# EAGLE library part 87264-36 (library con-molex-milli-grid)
RECEPTACAL
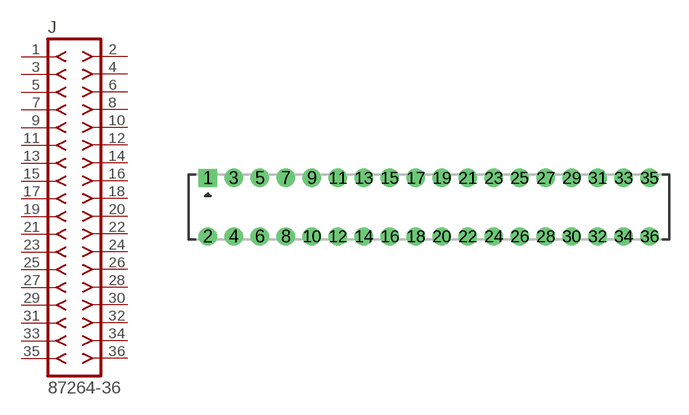
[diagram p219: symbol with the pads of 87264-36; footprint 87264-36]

Designator prefix J

## 87264-36  [87264-36]
1  1  pas
2  2  pas
3  3  pas
4  4  pas
5  5  pas
6  6  pas
7  7  pas
8  8  pas
9  9  pas
10  10  pas
11  11  pas
12  12  pas
13  13  pas
14  14  pas
15  15  pas
16  16  pas
17  17  pas
18  18  pas
19  19  pas
20  20  pas
21  21  pas
22  22  pas
23  23  pas
24  24  pas
25  25  pas
26  26  pas
27  27  pas
28  28  pas
29  29  pas
30  30  pas
31  31  pas
32  32  pas
33  33  pas
34  34  pas
35  35  pas
36  36  pas

## Footprint 87264-36 (pad centres in mm)
RECEPTACAL Dual Row, Side Entry
drill 0.914 square: 1 -17,2.25
drill 0.914: 2 -17,-2.25; 3 -15,2.25; 4 -15,-2.25; 5 -13,2.25; 6 -13,-2.25; 7 -11,2.25; 8 -11,-2.25; 9 -9,2.25; 10 -9,-2.25; 11 -7,2.25; 12 -7,-2.25; 13 -5,2.25; 14 -5,-2.25; 15 -3,2.25; 16 -3,-2.25; 17 -1,2.25; 18 -1,-2.25; 19 1,2.25; 20 1,-2.25; 21 3,2.25; 22 3,-2.25; 23 5,2.25; 24 5,-2.25; 25 7,2.25; 26 7,-2.25; 27 9,2.25; 28 9,-2.25; 29 11,2.25; 30 11,-2.25; 31 13,2.25; 32 13,-2.25; 33 15,2.25; 34 15,-2.25; 35 17,2.25; 36 17,-2.25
